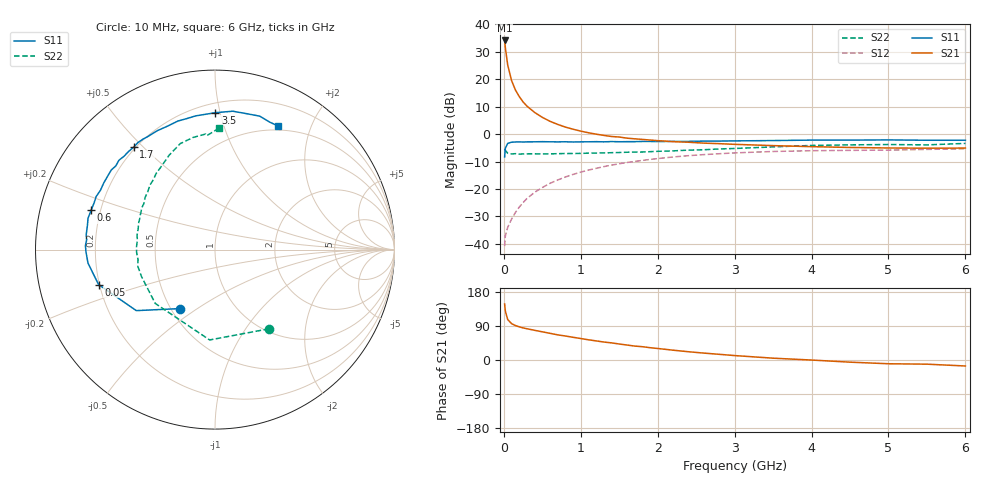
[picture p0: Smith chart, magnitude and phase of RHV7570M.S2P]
! SIEMENS Small Signal Semiconductors
! BFR106
! Si NPN RF Bipolar Junction Transistor in SOT23
! VCE = 0.75 V  IC = 70 mA
! Common Emitter S-Parameters:  August  1996
# GHz  S  MA  R  50
!  f  S11  S21  S12  S22
! GHz  MAG  ANG  MAG  ANG  MAG  ANG  MAG  ANG
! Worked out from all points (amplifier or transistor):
!   36 points, 10 MHz to 6 GHz, reference 50 ohm
!   highest |S21| = 34.1 dB at 10 MHz (marker M1)
!   |S21| within 3 dB of that: start of sweep to 21.44 MHz
!   unconditionally stable (mu >= 1): 84.57 MHz to end of sweep
!   at 250 MHz: K = 1.29, MAG = 15.1 dB, |S12| = -25.0 dB
!   at 1.4 GHz: K = 1.19, MAG = 2.5 dB, |S12| = -11.3 dB
!   at 6 GHz: K = 1.04, MAG = -1.0 dB, |S12| = -5.3 dB
!   S11 on the Smith chart (normalised r, x): 10 MHz: 0.55, -0.43; 50 MHz: 0.20, -0.14; 600 MHz: 0.16, +0.15; 1.7 GHz: 0.19, +0.47; 3.5 GHz: 0.26, +0.97; 6 GHz: 0.45, +1.54
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0.01  0.3836 -121.0  50.77 147.8  0.0091 62.8  0.5342 -55.7
0.02  0.5548 -142.2  37.2 128.7  0.0141 51.1  0.5042 -93.4
0.05  0.6773 -163.3  18.25 106.9  0.02 48.4  0.4482 -138.0
0.1  0.7115 -173.9  9.488 96.0  0.0282 57.1  0.4361 -159.9
0.15  0.7188 -178.9  6.391 91.0  0.0373 62.9  0.4401 -167.9
0.2  0.7223 178.2  4.84 87.5  0.0468 66.1  0.4325 -172.5
0.25  0.7171 175.7  3.855 84.7  0.0564 67.6  0.4351 -176.1
0.3  0.7224 173.6  3.241 82.5  0.0672 68.9  0.4371 -178.2
0.4  0.7235 169.2  2.482 78.3  0.0869 69.5  0.4374 178.0
0.5  0.7286 166.1  2.02 74.4  0.1064 68.9  0.4362 174.8
0.6  0.7242 162.4  1.711 70.4  0.1268 67.9  0.4365 172.5
0.7  0.7222 158.6  1.502 66.4  0.146 66.5  0.4405 170.2
0.8  0.725 155.9  1.343 63.3  0.1656 64.7  0.4429 167.6
1.1  0.7243 145.9  1.058 53.3  0.2212 59.4  0.4502 161.4
1.3  0.7231 139.8  0.947 47.4  0.2559 55.3  0.4543 157.0
1.7  0.7287 128.5  0.821 36.8  0.3179 47.5  0.4708 148.9
2.2  0.7363 115.9  0.729 25.9  0.3832 37.6  0.4946 139.1
3.5  0.763 89.8  0.617 4.8  0.4827 15.5  0.5848 115.9
4.5  0.7777 76.7  0.571 -5.7  0.5057 2.3  0.6368 101.0
5  0.7841 71.5  0.559 -9.9  0.511 -2.9  0.6461 94.6
5.5  0.773 66.8  0.554 -11.0  0.5266 -5.4  0.6366 94.1
6  0.7729 62.9  0.557 -15.8  0.541 -11.4  0.6773 88.1
